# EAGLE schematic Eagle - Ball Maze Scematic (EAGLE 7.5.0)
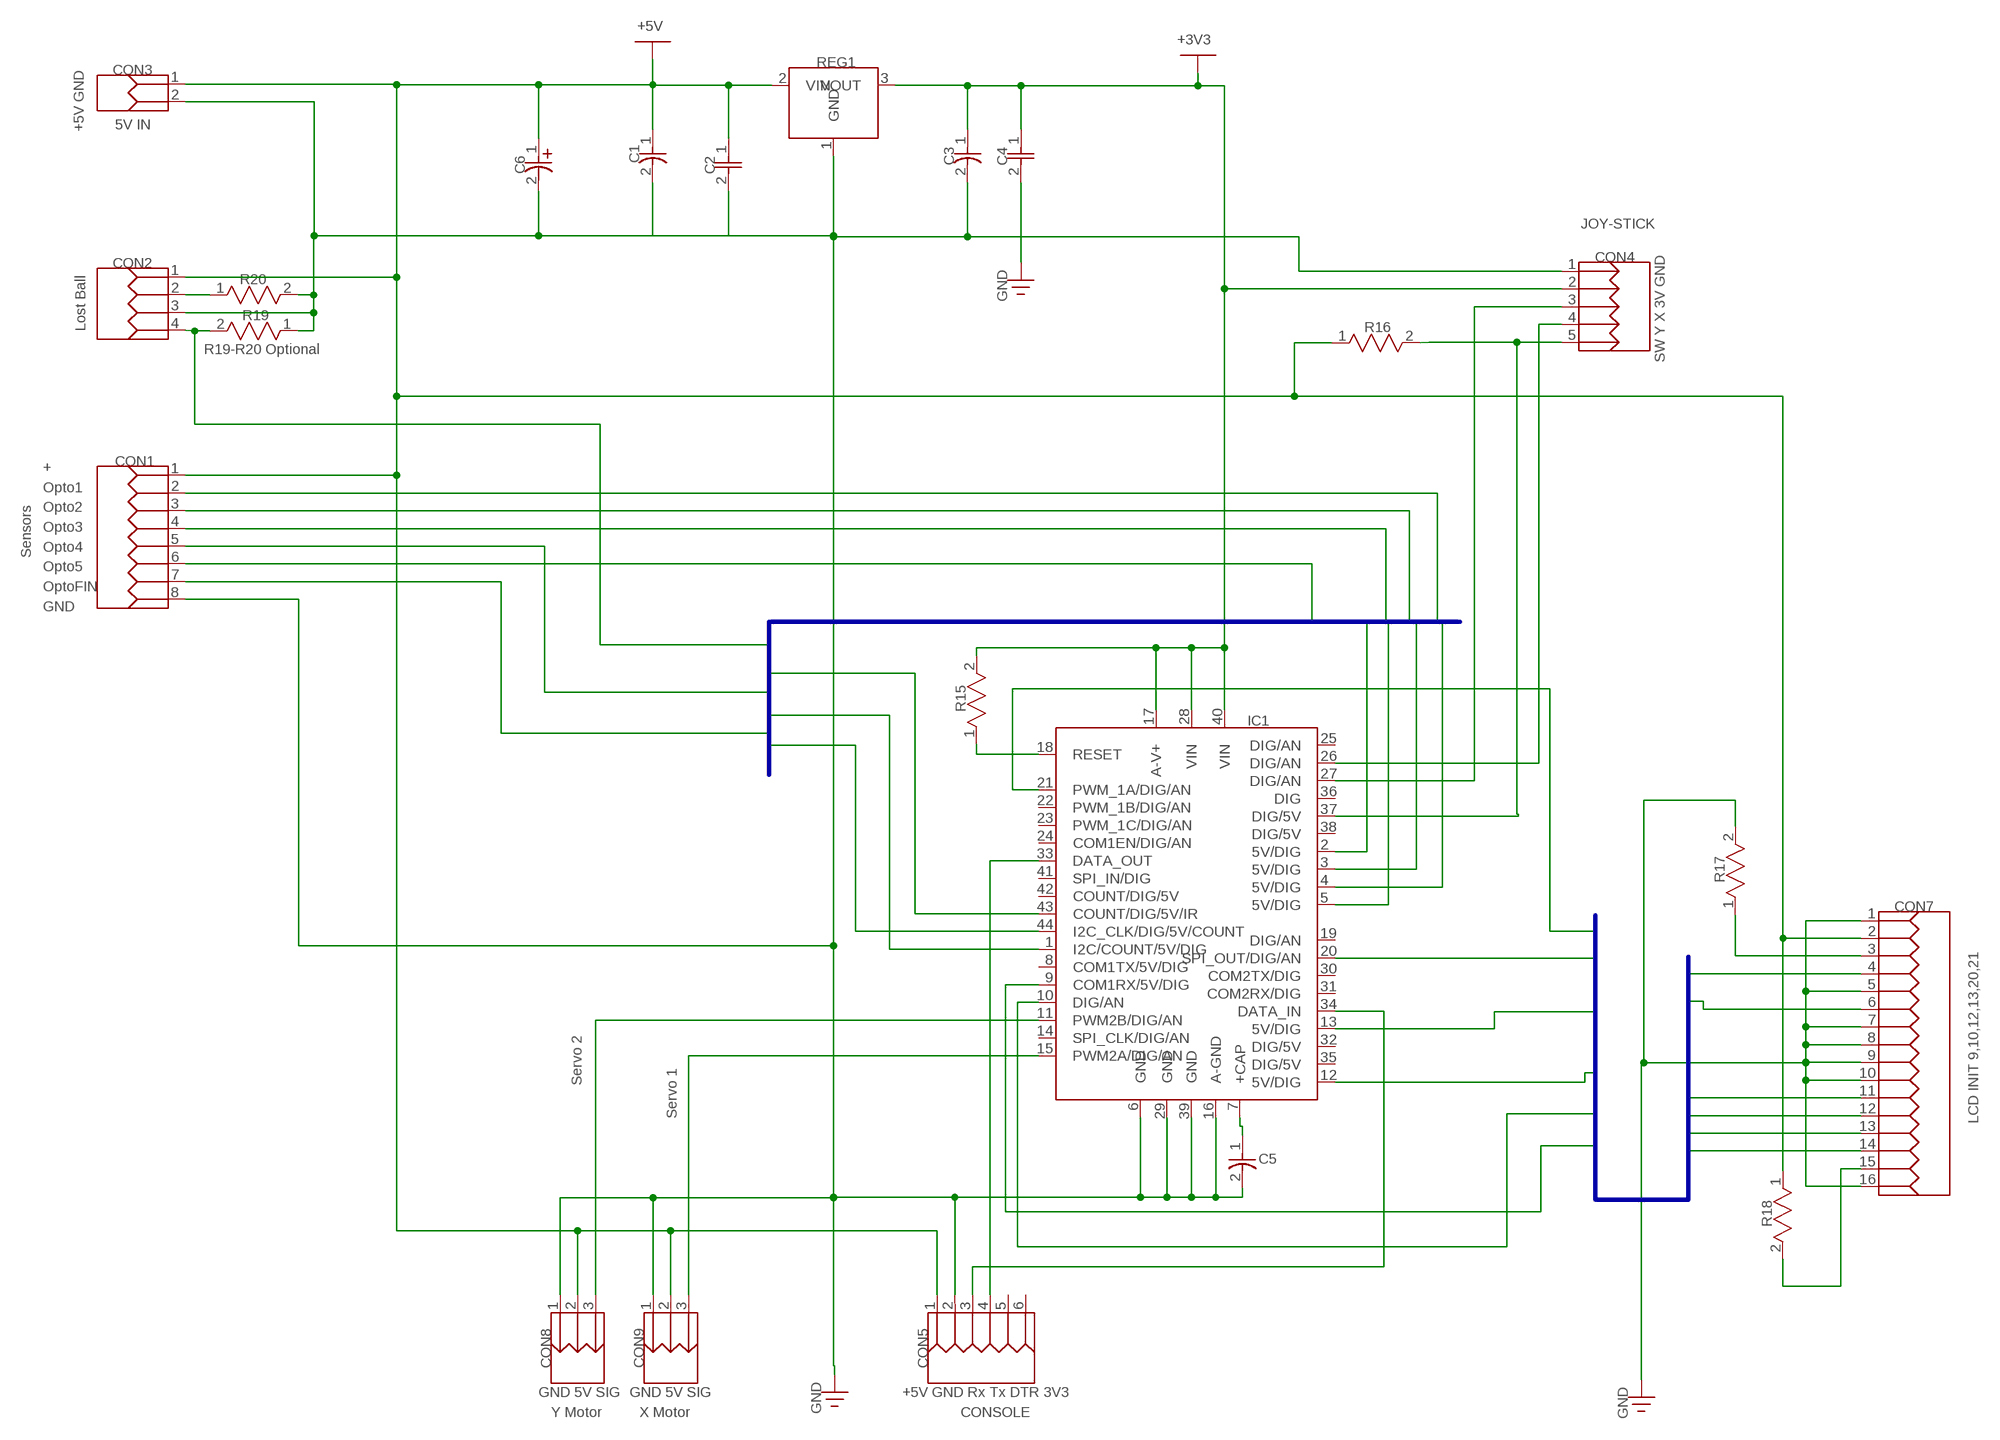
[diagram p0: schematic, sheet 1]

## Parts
C1  10uF  CAP_NONPOLARIZED  [CAP_1206]
C2  100n  CAP_NONPOLARIZED_3  [CAP_1206]
C3  10uF  CAP_NONPOLARIZED  [CAP_1206]
C4  100n  CAP_NONPOLARIZED_3  [CAP_1206]
C5  47uF 16V X5R  CAP  [CAP_1206]
C6  C220UF  [CAPAE-8.35X8.35H6.2]
CON1  51022-0800  [CON8M]
CON2  51022-0400  [CON4M]
CON3  DF4-2P-2C  [CON2M]
CON4  644456-5  [HDR-1X5T/2.54/12X2]
CON5  51022-0600  [CON6F]
CON7  HDRF-1X16  [CON16M]
CON8  644456-3  [HDR-1X3T/2.54/7X2]
CON9  644456-3  [HDR-1X3T/2.54/7X2]
IC1  PIC32MX-D/A_44PINS  [QFP45P80_1200X1200X160L60X37T220L]
R15  10K  RES  [RES_1206]
R16  1K  RES  [RES_1206]
R17  1K8  RES  [RES_1206]
R18  1K8  RES  [RES_1206]
R19  10K  RES  [RES_1206]
R20  150R  RES  [RES_1206]
REG1  MCP1700T-33  [TO92-127P520H787-3_AP3_STA]

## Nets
D4: CON7.11 IC1.9(COM1RX/5V/DIG)
D5: CON7.12 IC1.10(DIG/AN)
D6: CON7.13 IC1.12(5V/DIG)
D7: CON7.14 IC1.13(5V/DIG)
EN: CON7.6 IC1.21(PWM_1A/DIG/AN)
Net_0: C1.2 C2.2 C3.2 C4.2 C5.2 C6.2(MINUS) CON1.8 CON2.3 CON3.2 CON4.1 CON5.2 CON7.1 CON7.5 CON7.7 CON7.8 CON7.9 CON7.10 CON7.16 CON8.1 CON9.1 IC1.6(GND) IC1.16(A-GND) IC1.29(GND) IC1.39(GND) R17.2(B) R19.1(A) R20.2(B) REG1.1(GND) ; supply symbol labelled GND
Net_1: C3.1 C4.1 CON4.2 IC1.17(A-V+) IC1.28(VIN) IC1.40(VIN) R15.2(B) REG1.3(VOUT) ; supply symbol labelled +3V3
Net_2: CON4.4 IC1.26(DIG/AN)
Net_4: C1.1 C2.1 C6.1(PLUS) CON1.1 CON2.1 CON3.1 CON5.1 CON7.2 CON8.2 CON9.2 R16.1(A) R18.1(A) REG1.2(VIN) ; supply symbol labelled +5V
Net_14: CON5.3 IC1.34(DATA_IN)
Net_16: CON5.4 IC1.33(DATA_OUT)
Net_22: CON7.3 R17.1(A)
Net_23: CON4.3 IC1.27(DIG/AN)
Net_24: IC1.18(RESET) R15.1(A)
Net_27: C5.1 IC1.7(+CAP)
Net_29: CON4.5 IC1.37(DIG/5V) R16.2(B)
Net_31: CON2.2 R20.1(A)
Net_36: CON7.15 R18.2(B)
Net_42: CON9.3 IC1.15(PWM2A/DIG/AN)
Net_43: CON8.3 IC1.11(PWM2B/DIG/AN)
Opto1: CON1.2 IC1.4(5V/DIG)
Opto2: CON1.3 IC1.3(5V/DIG)
Opto3: CON1.4 IC1.2(5V/DIG)
Opto4: CON1.5 IC1.1(I2C/COUNT/5V/DIG)
Opto5: CON1.6 IC1.5(5V/DIG)
OptoFIN: CON1.7 IC1.44(I2C_CLK/DIG/5V/COUNT)
OptoLOST: CON2.4 IC1.43(COUNT/DIG/5V/IR) R19.2(B)
RS: CON7.4 IC1.20(SPI_OUT/DIG/AN)
Unconnected: CON5.5 CON5.6 IC1.8(COM1TX/5V/DIG) IC1.14(SPI_CLK/DIG/AN) IC1.19(DIG/AN) IC1.22(PWM_1B/DIG/AN) IC1.23(PWM_1C/DIG/AN) IC1.24(COM1EN/DIG/AN) IC1.25(DIG/AN) IC1.30(COM2TX/DIG) IC1.31(COM2RX/DIG) IC1.32(DIG/5V) IC1.35(DIG/5V) IC1.36(DIG) IC1.38(DIG/5V) IC1.41(SPI_IN/DIG)

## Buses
OptoFIN,OptoLOST,Opto2,Opto3,Opto4,Opto5,Opto1
D4,D5,D6,D7,EN,RS

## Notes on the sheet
- +5V
- +3V3
- +5V GND | REG1
- CON3
- 5V IN
- C1 | C3 | C4
- C6 | C2
- JOY-STICK
- CON4
- CON2
- R20
- GND
- R19
- Lost Ball | R16
- R19-R20 Optional
- SW Y X 3V GND
- +
  Opto1
  Opto2
  Opto3
  Opto4
  Opto5
  OptoFIN
  GND
- CON1
- Sensors
- R15
- IC1
- R17
- CON7
- Servo 2
- Servo 1
- LCD INIT 9,10,12,13,20,21
- C5
- R18
- CON8 | CON9 | CON5
- GND 5V SIG | GND 5V SIG | +5V GND Rx Tx DTR 3V3
- Y Motor | X Motor | CONSOLE
- GND
- GND

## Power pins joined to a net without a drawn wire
COUNT/DIG/5V: IC1.42(COUNT/DIG/5V)

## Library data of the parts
C1 C3 = common:CAP_NONPOLARIZED
C2 C4 = common:CAP_NONPOLARIZED_3; DESCRIPTION: Non-polarized
C5 = common:CAP
C6 = common:C220UF
CON1 = common:51022-0800; DATASHEET: http://datasheets.diptrace.com/con_board_in/510221400_sd.pdf; MANUFACTURER: Molex
CON2 = common:51022-0400; DATASHEET: http://datasheets.diptrace.com/con_board_in/510221400_sd.pdf; MANUFACTURER: Molex
CON3 = common:DF4-2P-2C; DATASHEET: http://datasheets.diptrace.com/con_board_in/DF4.pdf; MANUFACTURER: Hirose
CON4 = common:644456-5; DATASHEET: http://datasheets.diptrace.com/con_headers/ENG_CD_644456_D2.pdf; MANUFACTURER: TE Connectivity
CON5 = common:51022-0600; DATASHEET: http://datasheets.diptrace.com/con_board_in/510221400_sd.pdf; MANUFACTURER: Molex
CON7 = common:HDRF-1X16
CON8 CON9 = common:644456-3; DATASHEET: http://datasheets.diptrace.com/con_headers/ENG_CD_644456_D2.pdf; MANUFACTURER: TE Connectivity
IC1 = common:PIC32MX-D/A_44PINS
R15 R19 = common:RES
R16-R18 R20 = common:RES; VALUE: 10K
REG1 = common:MCP1700T-33; DATASHEET: http://datasheets.diptrace.com/microchip/20001826d.pdf; MANUFACTURER: Microchip; PART_NUMBER_(DIGI-KEY): MCP1700T3302EMBDKR-ND; UNIQUE_NAME: MICROCHIP_C04-029C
